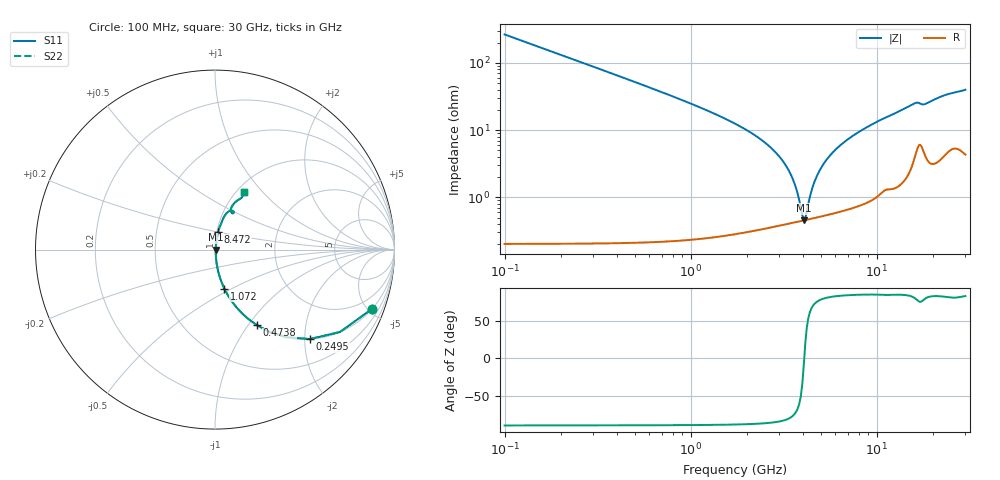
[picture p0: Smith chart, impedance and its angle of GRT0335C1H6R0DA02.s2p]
!Murata Part Number: GRT0335C1H6R0DA02
!These Parameters are Measured in Series Mode Connection
!Data Generated on Jun 19, 2026
!  o--ll--o
!Port1  Port2
!  o------o
!Operation Temp=25[degC], DC Bias Voltage=0[V]
!Freq. Start=100[MHz] Stop=30[GHz] 401[Steps]
# Hz S RI R 50
!Freq.(Hz) S11(Real) S11(Imag) S21(Real) S21(Imag) S12(Real) S12(Imag) S22(Real) S22(Imag)
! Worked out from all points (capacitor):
!   401 points, 100 MHz to 30 GHz, reference 50 ohm
!   read as one part in series: C = 6 pF near 249.5 MHz
!   lowest |Z| = 458 mohm at 4.062 GHz (marker M1)
!   series resonance near 4.081 GHz, so ESL is about 250 pH
!   S11 on the Smith chart (normalised r, x): 100 MHz: 1.00, -5.30; 249.5 MHz: 1.00, -2.12; 473.8 MHz: 1.00, -1.10; 1.072 GHz: 1.00, -0.46; 8.472 GHz: 1.02, +0.21; 30 GHz: 1.09, +0.79
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1e8  0.8752 -0.3301  0.1248 0.3301  0.1248 0.3301  0.8752 -0.3301
2.495e8  0.5286 -0.4982  0.4714 0.4982  0.4714 0.4982  0.5286 -0.4982
4.7375e8  0.2345 -0.4218  0.7655 0.4218  0.7655 0.4218  0.2345 -0.4218
6.98e8  0.121 -0.3232  0.879 0.3232  0.879 0.3232  0.121 -0.3232
1.07175e9  0.0522 -0.2174  0.9478 0.2174  0.9478 0.2174  0.0522 -0.2174
1.894e9  0.0146 -0.1074  0.9854 0.1074  0.9854 0.1074  0.0146 -0.1074
3.16475e9  0.00497 -0.0328  0.995 0.0328  0.995 0.0328  0.00497 -0.0328
3.5385e9  0.00449 -0.0182  0.9955 0.0182  0.9955 0.0182  0.00449 -0.0182
3.91225e9  0.00445 -0.00537  0.9956 0.00537  0.9956 0.00537  0.00445 -0.00537
4.06175e9  0.00452 -0.000595  0.9955 0.000595  0.9955 0.000595  0.00452 -0.000595
4.21125e9  0.00464 0.004  0.9954 -0.004  0.9954 -0.004  0.00464 0.004
4.4355e9  0.00488 0.0106  0.9951 -0.0106  0.9951 -0.0106  0.00488 0.0106
4.65975e9  0.0052 0.0169  0.9948 -0.0169  0.9948 -0.0169  0.0052 0.0169
5.10825e9  0.00604 0.0287  0.994 -0.0287  0.994 -0.0287  0.00604 0.0287
5.6315e9  0.0073 0.0415  0.9927 -0.0415  0.9927 -0.0415  0.0073 0.0415
6.379e9  0.00951 0.0583  0.9905 -0.0583  0.9905 -0.0583  0.00951 0.0583
8.472e9  0.018 0.1  0.982 -0.1  0.982 -0.1  0.018 0.1
1.01165e10  0.0274 0.1294  0.9726 -0.1294  0.9726 -0.1294  0.0274 0.1294
1.505e10  0.0698 0.2079  0.9302 -0.2079  0.9302 -0.2079  0.0698 0.2079
2.005825e10  0.0954 0.2426  0.9046 -0.2426  0.9046 -0.2426  0.0954 0.2426
2.50665e10  0.1429 0.2847  0.8571 -0.2847  0.8571 -0.2847  0.1429 0.2847
3e10  0.1626 0.3185  0.8374 -0.3185  0.8374 -0.3185  0.1626 0.3185
